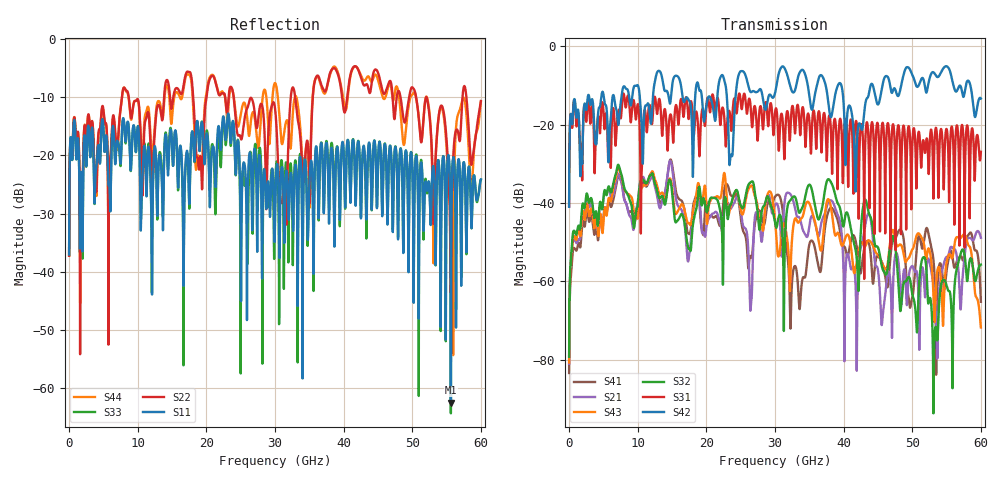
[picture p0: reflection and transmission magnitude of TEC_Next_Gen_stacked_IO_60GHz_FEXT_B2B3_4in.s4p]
!! CHANNEL DESCRIPTION:  Next Generation 28Gbps Press-fit Stacked I/O Connector
!!  with 4" 5-6-5 Megtron 6 Stripline trace on host side and 1.25" 7-5-7 Megtron 6 Microstrip trace on plug side
!! HOST PCB DESCRIPTION:  PCB thickness 3.425 mm
!!  26 Layer Board, 15 GND planes, 4 Layer route-out on Layers 7,11,17,21, 8mil stub on vias
!!  Pairs on following layers
!!  Layer 07 - A02A03 A14A15 D05D06
!!  Layer 11 - D020D3 C05C06 D14D15
!!  Layer 17 - C02C03 B05B06 C14C15
!!  Layer 21 - B02B03 A05A06 B14B15
!! CONNECTOR DESCRIPTION:  Next Generation 28Gbps Press-fit Stacked I/O Connector
!! PLUG-IN CARD DESCRIPTION:  PCB thickness 1mm thick
!!  6 Layer Board, 4 GND planes, 0.35 x 1.4mm mating pads
!!  Micro-strip diff traces referenced to GND plane 3mils down, 2nd GND plane 17mils from top of board
!!  PCB GND planes are symmetric
!! MODEL DESCRIPTION: TE Connectivity S-parameter model produced from Macro-model, Extracted .s4p FEXT (Victim B05B06 - Aggressor B02B03)
!! MODEL DATE: 5/15/2014 CR32f, FPR23
!! MODEL STATUS: Developmental
!! MODEL GEOMETRY: 4 Rows - Rows A, B, C, D. 3 pairs in each row, 12 total pairs
!! MODEL FREQUENCY RANGE: DC to 60 GHz in 10 MHz frequency steps
!! MODEL EDGE RATE LIMITATION: 8.33 ps (Using conservative 0.5/Fmax rule of thumb)
!! TIME-DOMAIN TRANSFORM CAUTIONS:
!! 1.) Do not simulate transient edge rates faster than the number listed above.  Edge
!!  rates faster than this number contain significant spectral content at frequencies
!!  above the model's highest frequency.
!! 2.) Even when simulating edge rates that are slower than the number listed above, be
!!  aware that the best time resolution possible with a direct iFFT is (1 / 2Fmax).
!!  As a result, time resolution is typically not adequate for most time-domain
!!  simulations unless tricks such as frequency-domain zero-padding and windowing are
!!  used to minimize leakage and aliasing.
!! 3.) Because the model has a uniform frequency step, a direct iFFT will result in an
!!  impulse that that has a time length given by either (1 / Fstep) or (1 / 2Fstep),
!!  depending on the transform being used.  Care has been taken in selecting the
!!  frequency step to ensure a settled impulse response for the model.  Therefore,
!!  convolution with the model's impulse response should present no issues.  However,
!!  if directly concatenating s-parameter models in the frequency domain a user must
!!  either interpolate necessary interim frequencies or complete impulse response
!!  zero-padding.  Impulse response zero-padding is more difficult, but more accurate.
!! PORT DEFINITIONS:
!! Port  1  ----->  Host B02		B05 Module <-----  Port  2
!! Port  3  ----->  Host B03		B06 Module <-----  Port  4
! Touchstone data
! Created: 29-Sep-2014 by IdEM R2011 (7.0.3)
# Hz S MA R 50
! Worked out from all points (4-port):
!   6000 points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, 10 MHz to 60 GHz, reference 50 ohm
!   strongest paths, dB at 10 MHz, 15.01 GHz, 30.01 GHz, 45.01 GHz, 60 GHz:
!     S42: -41.0, -10.1, -12.0, -14.9, -13.4
!     S31: -40.8, -20.1, -17.0, -20.2, -27.0
!     S32: -79.2, -37.2, -45.0, -51.3, -55.7
!     S43: -80.7, -36.1, -44.2, -53.2, -71.7
!     S21: -81.0, -30.9, -40.6, -57.2, -48.9
!     S41: -83.4, -30.2, -38.4, -53.5, -65.2
!   lowest |S11| = -62.6 dB at 55.63 GHz (marker M1), VSWR 1.00, Z = 49.9 - j0.0338 ohm
!   |S11| at or under -10 dB: start of sweep to end of sweep
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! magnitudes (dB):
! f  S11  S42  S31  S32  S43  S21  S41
! 10 MHz  -37.1  -41.0  -40.8  -79.2  -80.7  -81.0  -83.4
! 7.2 GHz  -18.1  -20.0  -16.6  -30.3  -30.8  -32.6  -33.0
! 26.47 GHz  -20.9  -11.7  -15.8  -34.7  -35.6  -66.7  -53.6
! 31.46 GHz  -28.3  -5.8  -24.6  -49.6  -45.8  -39.0  -47.9
! 44.71 GHz  -21.8  -13.6  -23.1  -51.1  -52.7  -56.1  -54.3
! 55.63 GHz  -62.6  -7.2  -21.6  -64.8  -53.6  -51.2  -52.1
! 60 GHz  -24.1  -13.4  -27.0  -55.7  -71.7  -48.9  -65.2
